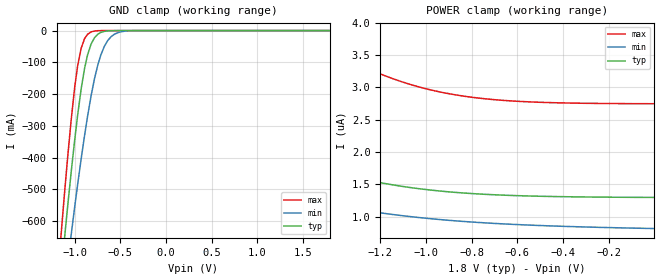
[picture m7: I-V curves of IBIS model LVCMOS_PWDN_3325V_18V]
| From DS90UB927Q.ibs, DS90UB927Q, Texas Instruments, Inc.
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|   Model
[Model] LVCMOS_PWDN_3325V_18V
Model_type Input
Vinh = 1.17V
Vinl = 0.63V
C_comp   6.98pF   6.05pF   8.06pF
[Voltage Range]   1.8V   1.62V   1.98V
[Temperature Range]   25.0   130.0   -40.0
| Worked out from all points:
|   GND clamp passes 1 mA (typ) near -0.64 V on its own axis
[GND Clamp]
-1.8V     -2.96A     -2.635A    -3.228A
-1.147V   -756.8mA   -899mA     -630.1mA
-1.114V   -658.8mA   -819.6mA   -517.7mA
-1.076V   -548.3mA   -728.9mA   -393.4mA
-1.039V   -442.8mA   -640.4mA   -278.7mA
-968.4mV  -265.6mA   -483.8mA   -110.5mA
-892.8mV  -119mA     -330.1mA   -25.28mA
-822.6mV  -43.25mA   -207.4mA   -4.316mA
-747mV    -11.34mA   -107.3mA   -362.8uA
-676.8mV  -2.576mA   -49.95mA   -25.05uA
-493.2mV  -20.33uA   -3.719mA   -5.105uA
1.796V    1.295uA    0A         2.744uA
[POWER Clamp]
-1.8V     2.219uA    1.514uA    15.57uA
-1.67V    2.017uA    1.387uA    4.242uA
-1.525V   1.824uA    1.263uA    3.836uA
-1.417V   1.705uA    1.184uA    3.591uA
-1.309V   1.606uA    1.116uA    3.382uA
-1.201V   1.525uA    1.057uA    3.209uA
-1.087V   1.458uA    1.006uA    3.064uA
-909mV    1.385uA    943.9nA    2.907uA
-801mV    1.356uA    915.2nA    2.847uA
-687.6mV  1.335uA    890.8nA    2.805uA
-433.8mV  1.309uA    852.1nA    2.761uA
-1.8mV    1.295uA    814nA      2.746uA
